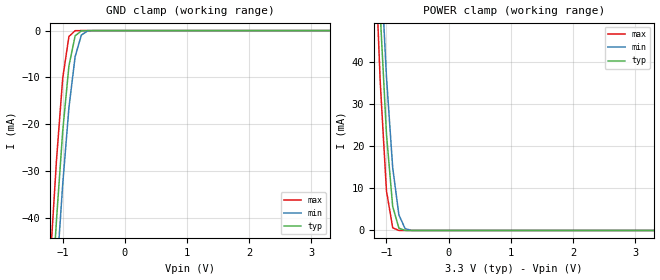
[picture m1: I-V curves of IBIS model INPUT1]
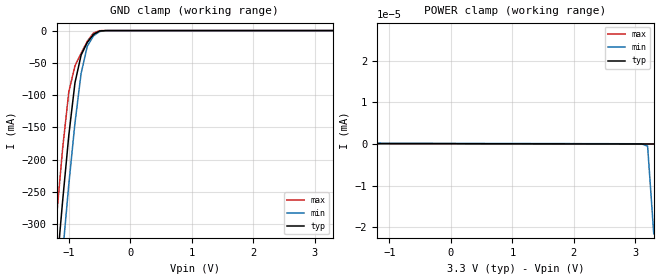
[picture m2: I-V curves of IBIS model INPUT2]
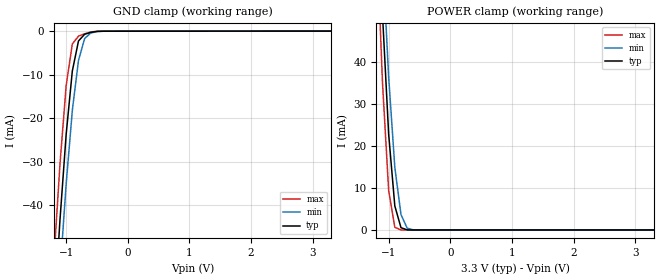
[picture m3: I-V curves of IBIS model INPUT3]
|   DIODES INCORPORATED
|   IBIS Model of PI6CG33201C
|   Product Family: 6CG
|   TQFN (ZD-24) Package
[IBIS Ver] 4.0
[Comment char] |_char
[File Name] pi6cg33201c_zd_reva.ibs
[File Rev] 1.0
[Source] File originated at Diodes Incorporated.
[Date] 04/02/2020
[Disclaimer] (C) Copyright DIODES INCORPORATED
   All rights reserved
  Diodes Incorporated hereby grants the user of
  this IBIS model a non-exclusive, nontransferable license to
  use this IBIS model under the following terms.
  This IBIS model is provided on an "AS IS" basis and Diodes
  makes absolutely no warranty with respect to the information
  contained herein. DIODES DISCLAIMS AND CUSTOMER WAIVES ALL
  WARRANTIES, EXPRESSED OR IMPLIED, INCLUDING WARRANTIES OF
  MERCHANTABILITY OR FITNESS FOR A PARTICULAR PURPOSE. The
  entire risk as to quality and performance is with the customer.
  Accordingly, in no event shall the company be liable for any
  damages, whether in contract or tort, including any lost
  profits or other incidental, consequential, exemplary, or
  punitive damages arising out of the use or application of the
  IBIS model provided in this package. Further, Diodes reserves
  the right to make changes without notice to any product herein
  to improve reliability, function, or design. Diodes does not
  convey any license under patent rights or any other intellectual
  property rights, including those of third parties.
  The user is granted this license only to use the IBIS model
  and is not granted rights to sell, load, rent, lease or license
  the IBIS model in whole or in part, or in modified form to anyone
  other than user. User may modify the IBIS model to suit its specific
  application but rights to derivative works and such modifications
  shall belong to Diodes.
  Diodes is not obligated to provide maintenance or support
  for the licensed IBIS model.
  Contact Diodes at ATTN: APPLICATION ENGINEERING / IBIS MODELS
  1545 Barber Ln. Milpitas, CA 95035
[Component] PI6CG33201C
[Manufacturer] Diodes Incorporated.
[Package]
| Variable   typ   min   max
R_pkg   0.03484ohm   0.02922ohm   0.04046ohm
L_pkg   0.78416nH   0.76828nH   0.80005nH
C_pkg   0.18668pF   0.17176pF   0.20160pF
[Pin]  signal_name   model_name   R_pin   L_pin   C_pin
1   XTAL_IN/CLK   INPUT1   0.04046   0.80005nH   0.20160pF
2   XTAL_OUT   OUTPUT   0.03484   0.78416nH   0.18668pF
3   VDD_OSC   POWER   0.02922   0.76828nH   0.17176pF
4   SADR/REFOUT   IO   0.02922   0.76828nH   0.17176pF
5   GND_REF   GND   0.03484   0.78416nH   0.18668pF
6   GND_DIG   GND   0.04046   0.80005nH   0.20160pF
7   VDD_DIG   POWER   0.04046   0.80005nH   0.20160pF
8   SCLK   INPUT2   0.03484   0.78416nH   0.18668pF
9   SDATA   IO_OS   0.02922   0.76828nH   0.17176pF
10   GND   GND   0.02922   0.76828nH   0.17176pF
11   VDD   POWER   0.03484   0.78416nH   0.18668pF
12   OE0#   INPUT3   0.04046   0.80005nH   0.20160pF
13   Q0+   HCSL_OUT   0.04046   0.80005nH   0.20160pF
14   Q0-   HCSL_OUT   0.03484   0.78416nH   0.18668pF
15   GNDA   GND   0.02922   0.76828nH   0.17176pF
16   VDDA   POWER   0.02922   0.76828nH   0.17176pF
17   Q1+   HCSL_OUT   0.03484   0.78416nH   0.18668pF
18   Q1-   HCSL_OUT   0.04046   0.80005nH   0.20160pF
19   OE1#   INPUT3   0.04046   0.80005nH   0.20160pF
20   VDD   POWER   0.03484   0.78416nH   0.18668pF
21   GND   GND   0.02922   0.76828nH   0.17176pF
22   PD#   INPUT4   0.02922   0.76828nH   0.17176pF
23   SS_SEL_TRI   INPUT5   0.03484   0.78416nH   0.18668pF
24   GND   GND   0.04046   0.80005nH   0.20160pF
| Models and submodels in the file (9): INPUT1 (Input), INPUT2 (Input), INPUT3 (Input), INPUT4 (Input), INPUT5 (Input), OUTPUT (Output), IO (I/O), IO_OS (I/O_open_sink), HCSL_OUT (Output)
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[Model] INPUT1
Model_type Input
Vinl = 825mV
Vinh = 2.75V
| variable   typ   min   max
C_comp   4.138pF   4.098pF   4.182pF
[Voltage Range]   3.3V   3.135V   3.465V
[GND Clamp Reference]   0.000V   0.000V   0.000V
[POWER Clamp Reference]   3.3V   3.135V   3.465V
[temperature range]   25   85   -40
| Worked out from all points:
|   GND clamp passes 1 mA (typ) near -0.79 V on its own axis
|   POWER clamp passes 1 mA (typ) near -0.81 V on its own axis
[GND Clamp]
| Voltage   I(typ)   I(min)   I(max)
-3.3V     -611mA     -617mA     -607mA
-1.2V     -62.2mA    -74.3mA    -49.3mA
-1.1V     -40.5mA    -52.6mA    -27.7mA
-1V       -21.5mA    -32.9mA    -10.2mA
-900mV    -7.54mA    -16.5mA    -1.27mA
-800mV    -1.13mA    -5.57mA    -24.2uA
-700mV    -53.2uA    -958uA     -202nA
-600mV    -1.35uA    -74.3uA    -1.53nA
3.3V      9.9pA      35.5pA     9.41pA
[POWER Clamp]   |Note: Vtable = Vcc - Voutput
| Voltage   I(typ)   I(min)   I(max)
-3.3V     1.02A      977mA      1.08A
-1.2V     86.3mA     99mA       71.7mA
-1.1V     51.3mA     65.5mA     35.1mA
-1V       22.8mA     36.4mA     9.39mA
-900mV    5.72mA     14.9mA     638uA
-800mV    544uA      3.68mA     8.25uA
-700mV    18.7uA     441uA      62.5nA
-600mV    428nA      26.6uA     460pA
3.3V      -9.9pA     -97pA      -9.41pA
[Model] INPUT2
Model_type Input
Vinl = 825mV
Vinh = 2.75V
| variable   typ   min   max
C_comp   2.377pF   2.375pF   2.379pF
[Voltage Range]   3.3V   3.135V   3.465V
[GND Clamp Reference]   0.000V   0.000V   0.000V
[POWER Clamp Reference]   3.3V   3.135V   3.465V
[temperature range]   25   85   -40
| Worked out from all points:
|   GND clamp passes 1 mA (typ) near -0.51 V on its own axis
|   POWER clamp passes 1 mA (typ) near -2.41 V on its own axis
[GND Clamp]
| Voltage   I(typ)   I(min)   I(max)
-3.3V     -3.1A      -3.15A     -3.08A
-1.3V     -486mA     -569mA     -402mA
-1.2V     -372mA     -455mA     -289mA
-1.1V     -263mA     -344mA     -182mA
-1V       -162mA     -238mA     -94.7mA
-900mV    -80.8mA    -143mA     -54.6mA
-800mV    -38mA      -66.3mA    -35.1mA
-700mV    -18.5mA    -24.4mA    -16.7mA
-600mV    -6.12mA    -8.27mA    -3.99mA
-500mV    -639uA     -1.47mA    -152uA
-400mV    -17.1uA    -85.9uA    -1.09uA
3.3V      65.7pA     151pA      64.9pA
[POWER Clamp]   |Note: Vtable = Vcc - Voutput
| Voltage   I(typ)   I(min)   I(max)
-3.3V     678mA      594mA      765mA
-2.2V     101nA      80.9nA     101nA
-2.1V     2.3nA      3.56nA     863pA
-2V       153pA      374pA      113pA
3.1V      4.4pA      39pA       7.18pA
3.2V      2.41pA     -514pA     5.21pA
3.3V      0A         -21.6nA    3.25pA
[Model] INPUT3
Model_type Input
Vinl = 825mV
Vinh = 2.75V
| variable   typ   min   max
C_comp   0.482pF   0.477pF   0.488pF
[Voltage Range]   3.3V   3.135V   3.465V
[GND Clamp Reference]   0.000V   0.000V   0.000V
[POWER Clamp Reference]   3.3V   3.135V   3.465V
[temperature range]   25   85   -40
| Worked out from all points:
|   GND clamp passes 1 mA (typ) near -0.72 V on its own axis
|   POWER clamp passes 1 mA (typ) near -0.81 V on its own axis
[GND Clamp]
| Voltage   I(typ)   I(min)   I(max)
-3.3V     -806mA     -784mA     -851mA
-1.2V     -65.6mA    -77.9mA    -52.7mA
-1.1V     -43.3mA    -55.5mA    -30.5mA
-1V       -23.7mA    -35.1mA    -12.5mA
-900mV    -9.15mA    -18.2mA    -2.93mA
-800mV    -2.24mA    -6.72mA    -1.13mA
-700mV    -702uA     -1.66mA    -594uA
-600mV    -266uA     -406uA     -185uA
-500mV    -41.5uA    -86.4uA    -13.4uA
3.3V      27.3uA     28.7uA     25.2uA
[POWER Clamp]   |Note: Vtable = Vcc - Voutput
| Voltage   I(typ)   I(min)   I(max)
-3.3V     1.02A      977mA      1.08A
-1.2V     86.3mA     99mA       71.7mA
-1.1V     51.3mA     65.5mA     35.1mA
-1V       22.8mA     36.4mA     9.39mA
-900mV    5.72mA     14.9mA     638uA
-800mV    544uA      3.68mA     8.25uA
-700mV    18.7uA     441uA      62.5nA
-600mV    428nA      26.6uA     460pA
3.3V      -9.9pA     -97pA      -9.41pA
